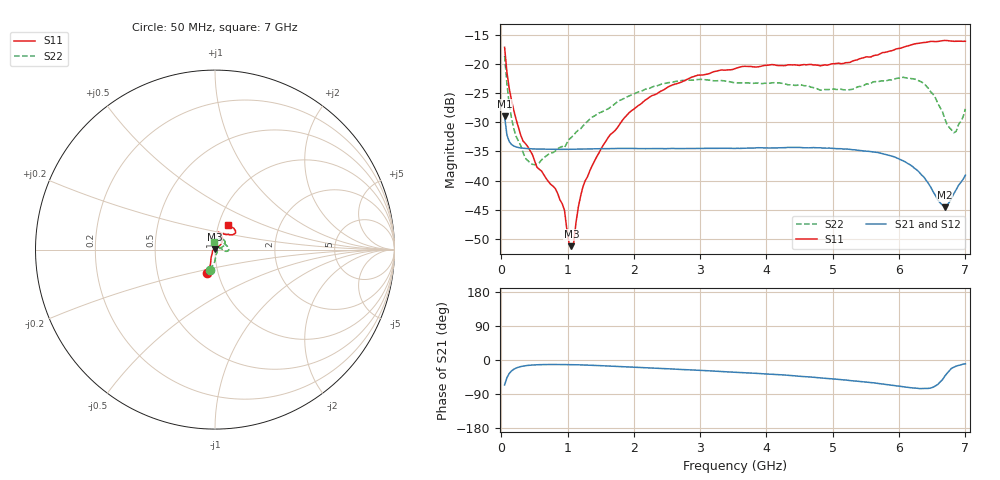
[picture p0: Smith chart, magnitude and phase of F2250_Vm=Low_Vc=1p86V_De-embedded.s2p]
! Integrated Device Technology
! Corporate Headquarters
! 6024 Silver Creek Valley Road
! San Jose, CA 95138  USA
! Phone:  1-408-284-8200
! Toll Free:  1-800-223-1366
! Webpage:  http://www.idt.com/
! Timing and RF Division
! 515 Groton Road, Suite 102
! Westford, MA 01886-6024
! Device:  F2250
! Description: Voltage Variable RF Attenuator
! Frequency:  50.0 -  6000.00 MHz
! Package:  3x3 mm Thin QFN Plastic Package: 16 pin
! Ports:  2 RF, 3 DC
!  Pin  1  = GND
!  Pin  2  = NC
!  Pin  3  = RF1  = Port 1
!  Pin  4  = NC
!  Pin  5  = GND
!  Pin  6  = GND
!  Pin  7  = GND
!  Pin  8  = GND
!  Pin  9  = NC
!  Pin 10  = RF2  = Port 2
!  Pin 11  = NC
!  Pin 12  = GND
!  Pin 13  = GND
!  Pin 14  = VCNTRL
!  Pin 15  = VDD
!  Pin 16  = VMODE
! Vcntrl:  1.860 Volts
! Vmode:  +0.000 Volts
! Vdd:  +3.30  Volts
! Current:  1.183 mA
! Data:  The device was measured on a the F2250 evaluation board which has
!  individual transmission lines to the RF pins.  Data was collected
!  using a calibrated network analyzer.  The evaluation board was
!  de-embedded using a TRL calibration technique.
!  The reference plane is the edge of the package pin.
! Misc:  SN 10
!  Action Tracker AT0258
! Date Measured:  2014-11-26
! Date:  2015-10-15  MJV
! Note:
!  Integrated Device Technology supplies this data as a sample of measured
!  data at the package pin for this product.  Your particular data for this
!  product may vary.
!  Data was taken at 25 degrees C.
!  Integrated Device Technology reserves the right to change this data at anytime.
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# GHz S dB R 50
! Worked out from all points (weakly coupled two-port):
!   201 points, 50 MHz to 7 GHz, reference 50 ohm
!   highest |S21| = -29.00 dB at 50 MHz (marker M1); lowest = -44.6 dB at 6.687 GHz (marker M2)
!   lowest |S11| = -51.2 dB at 1.058 GHz (marker M3), VSWR 1.01, Z = 49.9 + j0.237 ohm
!   |S11| at or under -10 dB: start of sweep to end of sweep
!   |S22| runs from -37.3 to -18.6 dB; largest |S21 - S12| = 5.9e-05
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0.05  -17.17 -108.5  -29.00 -65.6  -29.01 -65.6  -18.64 -103.4
0.08475  -21.43 -107.2  -32.18 -46.7  -32.18 -46.7  -23.44 -91.2
0.15425  -26.24 -116.3  -33.81 -28.8  -33.81 -28.8  -29.32 -82.4
0.29325  -32.22 -127.1  -34.41 -17.4  -34.41 -17.4  -34.02 -55.0
0.36275  -33.64 -138.5  -34.49 -15.1  -34.49 -15.1  -36.17 -37.2
0.5365  -37.68 -154.9  -34.59 -12.6  -34.60 -12.6  -37.16 -11.0
0.84925  -42.18 170.3  -34.64 -11.9  -34.64 -11.9  -34.56 5.9
0.9535  -45.08 170.1  -34.65 -12.0  -34.64 -12.1  -34.34 10.5
1.023  -50.80 142.8  -34.63 -12.2  -34.63 -12.2  -32.92 12.8
1.05775  -51.23 119.9  -34.63 -12.3  -34.63 -12.3  -32.59 14.4
1.0925  -50.62 85.3  -34.62 -12.4  -34.62 -12.4  -32.19 13.7
1.162  -44.54 54.4  -34.60 -12.7  -34.60 -12.7  -31.36 12.5
1.2315  -41.04 42.6  -34.59 -13.0  -34.58 -13.0  -30.64 11.9
1.6485  -32.08 41.4  -34.53 -15.9  -34.52 -15.9  -27.42 21.1
2.37825  -24.87 47.1  -34.51 -22.1  -34.51 -22.1  -23.65 30.7
3.525  -20.82 72.4  -34.49 -32.1  -34.48 -32.1  -23.25 58.3
4.7065  -20.19 72.3  -34.35 -45.5  -34.35 -45.5  -24.08 62.0
5.85325  -17.83 40.4  -35.69 -65.7  -35.69 -65.8  -22.75 6.8
6.3745  -16.34 41.3  -39.40 -75.3  -39.41 -75.3  -23.39 -7.8
6.68725  -16.00 48.8  -44.56 -43.3  -44.56 -43.1  -29.32 11.4
6.82625  -16.14 53.5  -42.22 -18.9  -42.18 -18.8  -31.80 50.6
7  -16.13 63.2  -39.07 -10.1  -39.03 -10.1  -27.71 96.4
